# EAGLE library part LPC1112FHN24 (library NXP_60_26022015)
32-bit ARM Cortex-M0 microcontroller; up to 64 kB flash and 8 kB SRAM The LPC1110/11/12/13/14/15 are a ARM Cortex-M0 based, low-cost 32-bit MCU family, designed for 8/16-bit microcontroller applications, offering performance, low power, simple instruction set and memory addressing together with reduced code size compared to existing 8/16-bit architectures. The LPC1110/11/12/13/14/15 operate at CPU frequencies of up to 50 MHz. The peripheral complement of the LPC1110/11/12/13/14/15 includes up to 64 kB of flash memory, up to 8 kB of data memory, one Fast-mode Plus I 2 C-bus interface, one RS-485/EIA-485 UART, up to two SPI interfaces with SSP features, four general purpose counter/timers, a 10-bit ADC, and up to 42 general purpose I/O pins. Remark: The LPC111x series consists of the LPC1100 series (parts LPC111x/101/201/301), LPC1100L series (parts LPC111x/002/102/202/302), and the LPC1100XL series (parts LPC111x/103/203/303/323/333). The LPC1100L and LPC1100XL series include the power profiles, a windowed watchdog timer, and a configurable open-drain mode. AAL Eindhoven MK
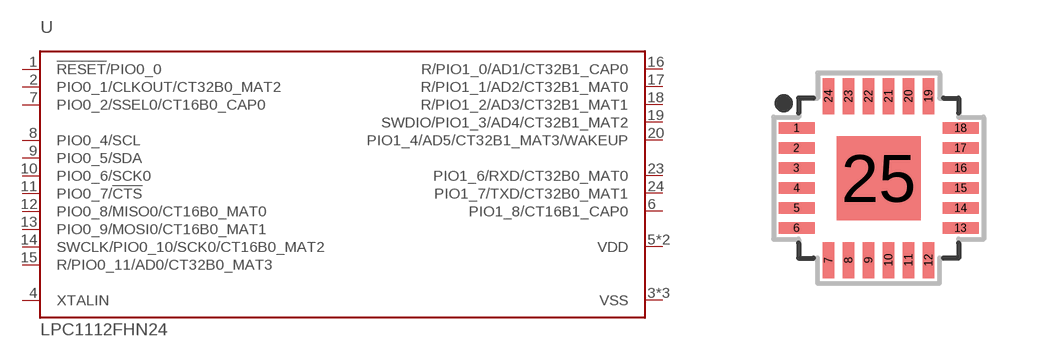
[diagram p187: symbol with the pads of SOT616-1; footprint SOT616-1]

Designator prefix U

## LPC1112FHN24/202 (ADC: 6; FLASH: 16kB; GPIO: 19; PWR_PROFILES: yes; SERIES: LPC1100L; SPI: 1; SRAM: 4kB)  [SOT616-1]
1  !RESET!/PIO0_0
2  PIO0_1/CLKOUT/CT32B0_MAT2
3  VSS  pwr
4  XTALIN  in
5  VDD  pwr
6  PIO1_8/CT16B1_CAP0
7  PIO0_2/SSEL0/CT16B0_CAP0
8  PIO0_4/SCL
9  PIO0_5/SDA
10  PIO0_6/SCK0
11  PIO0_7/!CTS!
12  PIO0_8/MISO0/CT16B0_MAT0
13  PIO0_9/MOSI0/CT16B0_MAT1
14  SWCLK/PIO0_10/SCK0/CT16B0_MAT2
15  R/PIO0_11/AD0/CT32B0_MAT3
16  R/PIO1_0/AD1/CT32B1_CAP0
17  R/PIO1_1/AD2/CT32B1_MAT0
18  R/PIO1_2/AD3/CT32B1_MAT1
19  SWDIO/PIO1_3/AD4/CT32B1_MAT2
20  PIO1_4/AD5/CT32B1_MAT3/WAKEUP
21  VSS  pwr
22  VDD  pwr
23  PIO1_6/RXD/CT32B0_MAT0
24  PIO1_7/TXD/CT32B0_MAT1
25  VSS  pwr

## Footprint SOT616-1 (pad centres in mm)
SOT616-1 HVQFN24: plastic thermal enhanced very thin quad flat package; no leads; 24 terminals; body 4 x 4 x 0.85 mm JEDEC: MO-220 IEC: -- JEITA: --
smd 0.9 x 0.29: 1 -2.05,1.25; 2 -2.05,0.75; 3 -2.05,0.25; 4 -2.05,-0.25; 5 -2.05,-0.75; 6 -2.05,-1.25; 13 2.05,-1.25; 14 2.05,-0.75; 15 2.05,-0.25; 16 2.05,0.25; 17 2.05,0.75; 18 2.05,1.25
smd 0.29 x 0.9: 7 -1.25,-2.05; 8 -0.75,-2.05; 9 -0.25,-2.05; 10 0.25,-2.05; 11 0.75,-2.05; 12 1.25,-2.05; 19 1.25,2.05; 20 0.75,2.05; 21 0.25,2.05; 22 -0.25,2.05; 23 -0.75,2.05; 24 -1.25,2.05
smd 2.1 x 2.1: 25 0,0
